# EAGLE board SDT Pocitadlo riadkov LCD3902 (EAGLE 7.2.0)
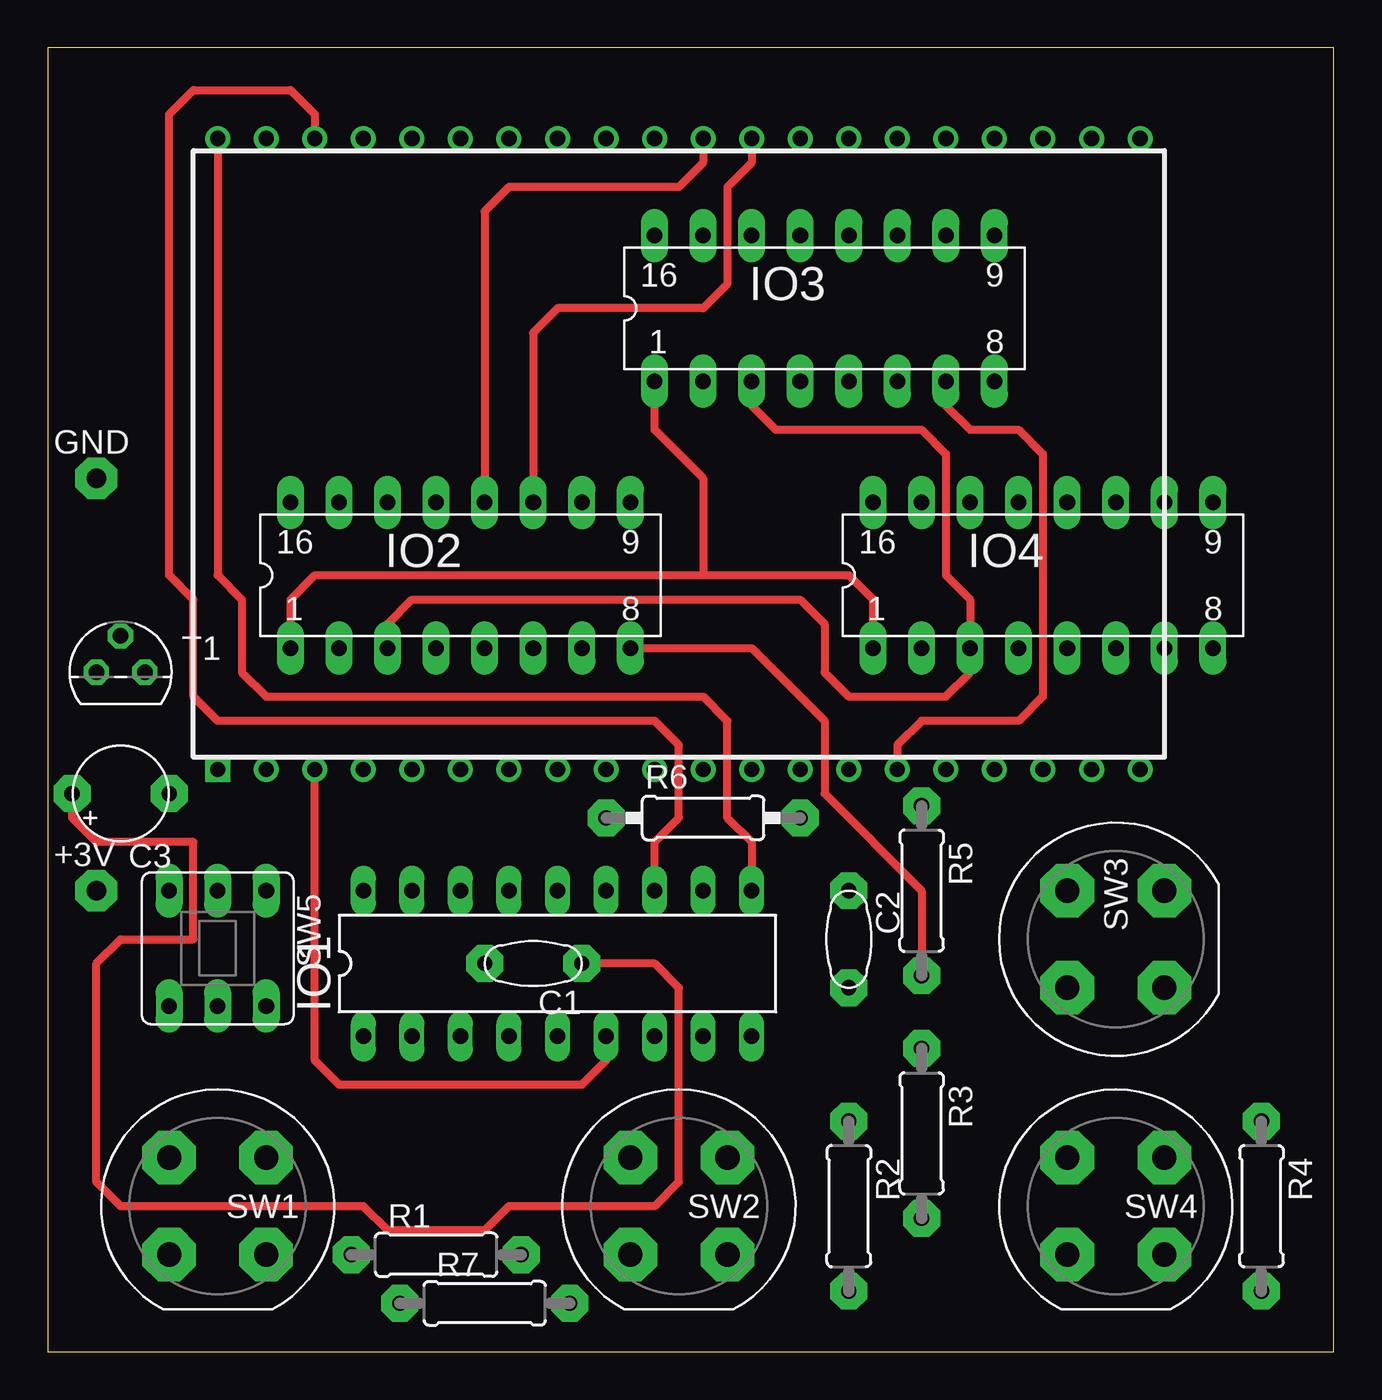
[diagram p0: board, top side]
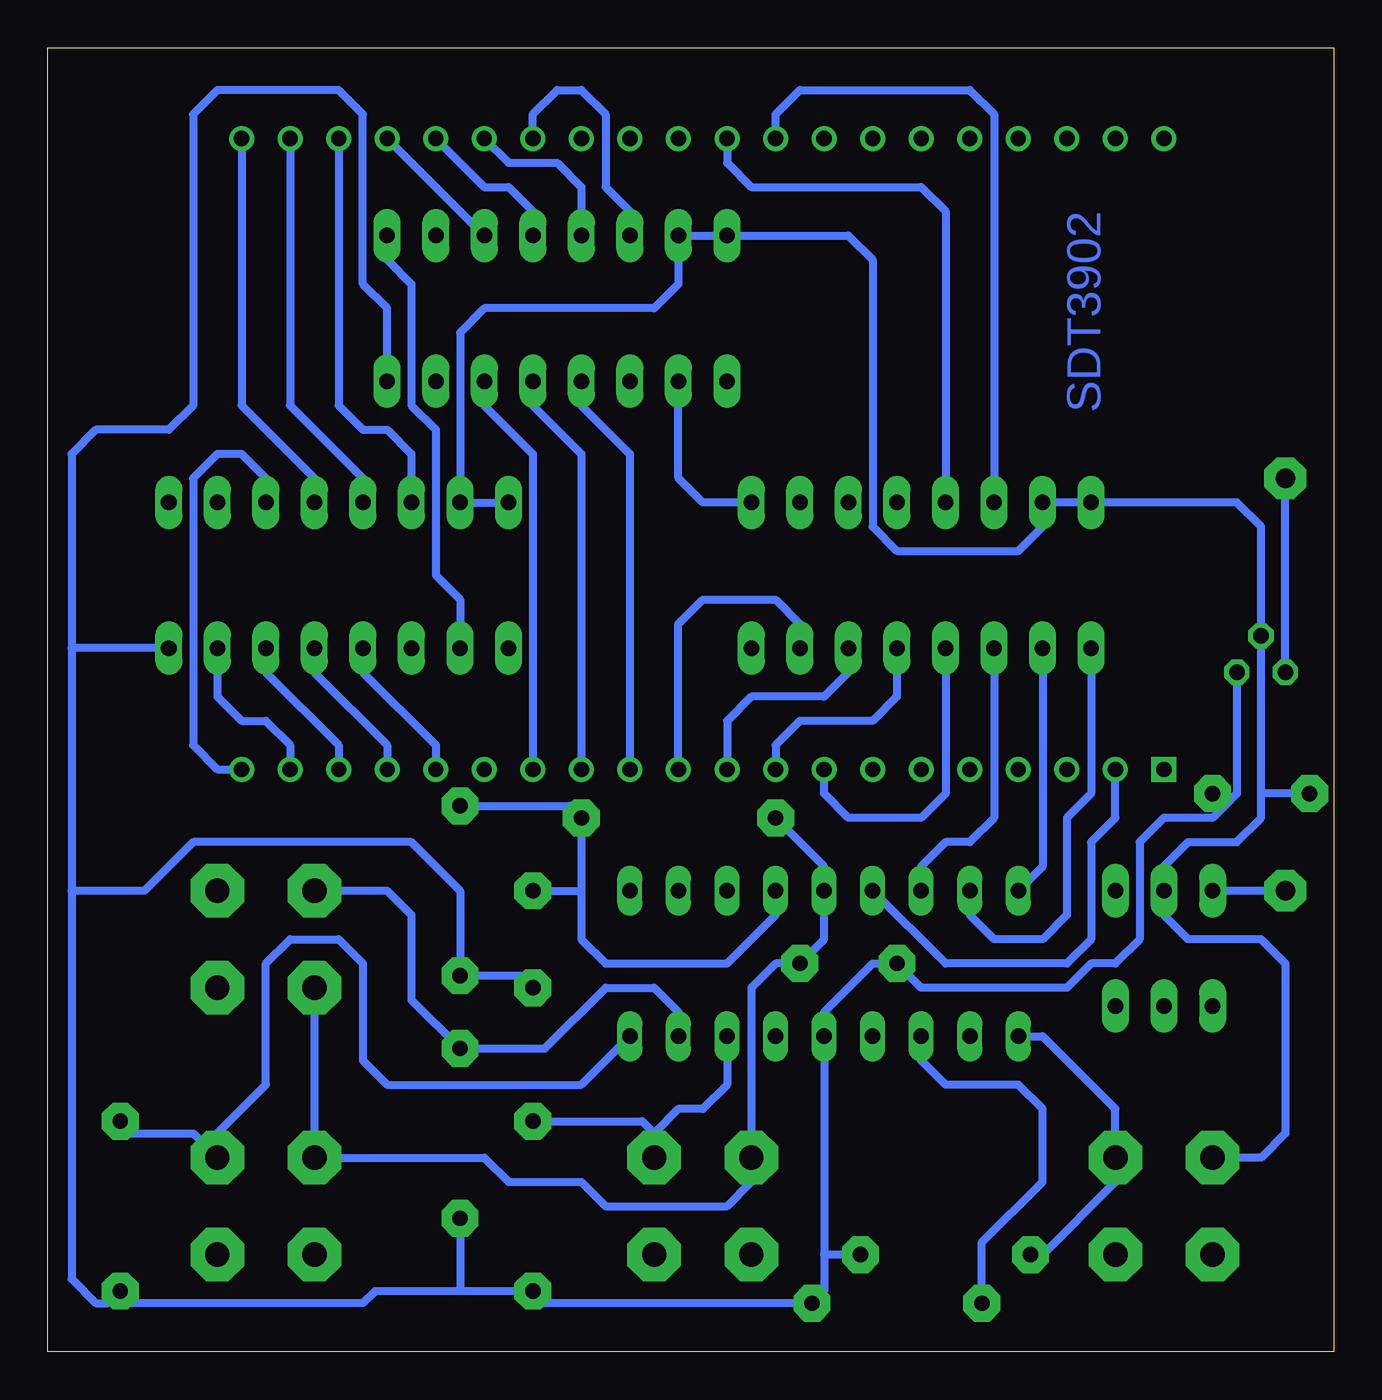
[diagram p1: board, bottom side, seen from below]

Size 67.29 x 68.25 mm. Coordinates in mm from the lower left corner, seen from the top.
Outline: 0,0 67.29,0 67.29,68.25 0,68.25 0,0
Copper layers (1*16): Top 0.035mm / dielectric 1.5mm / Bottom 0.035mm
Design rules "default": minimum track width 10mil, minimum drill 24mil, track to track 8mil, track to pad 8mil, pad to pad 8mil, via to via 8mil, smd to smd 8mil, copper to edge 40mil, drill to drill 8mil, minimum pad ring 10mil, minimum via ring 8mil, stop-mask expansion 4mil, vias tented up to drill 0mil, thermal gap 10mil

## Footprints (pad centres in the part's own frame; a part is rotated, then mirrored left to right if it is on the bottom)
PAD_1 = drill 1.016 pad 2.184 octagon: 1 0,0
KERAMICKY_RM5 = drill 0.8 pad 1.93 octagon: P$1 -2.54,0; P$2 2.54,0
ELEKTROLITICKY_RM5-5 = drill 0.8 pad 1.93 octagon: P$1 -2.54,0; P$2 2.54,0
4DR821_CN = drill 0.8 square: 1 -24.13,-16.51 | drill 0.8: 2 -21.59,-16.51; 3 -19.05,-16.51; 4 -16.51,-16.51; 5 -13.97,-16.51; 6 -11.43,-16.51; 7 -8.89,-16.51; 8 -6.35,-16.51; 9 -3.81,-16.51; 10 -1.27,-16.51; 11 1.27,-16.51; 12 3.81,-16.51; 13 6.35,-16.51; 14 8.89,-16.51; 15 11.43,-16.51; 16 13.97,-16.51; 17 16.51,-16.51; 18 19.05,-16.51; 19 21.59,-16.51; 20 24.13,-16.51; 21 24.13,16.51; 22 21.59,16.51; 23 19.05,16.51; 24 16.51,16.51; 25 13.97,16.51; 26 11.43,16.51; 27 8.89,16.51; 28 6.35,16.51; 29 3.81,16.51; 30 1.27,16.51; 31 -1.27,16.51; 32 -3.81,16.51; 33 -6.35,16.51; 34 -8.89,16.51; 35 -11.43,16.51; 36 -13.97,16.51; 37 -16.51,16.51; 38 -19.05,16.51; 39 -21.59,16.51; 40 -24.13,16.51
DIL18 = drill 0.813 long: 1 -8.89,-3.81; 2 -6.35,-3.81; 3 -3.81,-3.81; 4 -1.27,-3.81; 5 1.27,-3.81; 6 3.81,-3.81; 7 6.35,-3.81; 8 8.89,-3.81; 9 11.43,-3.81; 10 11.43,3.81; 11 8.89,3.81; 12 6.35,3.81; 13 3.81,3.81; 14 1.27,3.81; 15 -1.27,3.81; 16 -3.81,3.81; 17 -6.35,3.81; 18 -8.89,3.81
DIL16 = drill 0.813 pad 1.4 long: 1 -8.89,-3.81; 2 -6.35,-3.81; 3 -3.81,-3.81; 4 -1.27,-3.81; 5 1.27,-3.81; 6 3.81,-3.81; 7 6.35,-3.81; 8 8.89,-3.81; 9 8.89,3.81; 10 6.35,3.81; 11 3.81,3.81; 12 1.27,3.81; 13 -1.27,3.81; 14 -3.81,3.81; 15 -6.35,3.81; 16 -8.89,3.81
0207/7 = drill 0.8 pad 1.93 octagon: 1 -4.445,0; 2 4.445,0
0207/10 = drill 0.8 pad 1.93 octagon: 1 -5.08,0; 2 5.08,0
P-DT6 = drill 1.27 pad 2.8 octagon: 1 -2.54,-2.54; 1A -2.54,2.54; 2 2.54,-2.54; 2A 2.54,2.54
P-B170 = drill 0.813 pad 1.4 long: 1 0,5.08; 2 0,2.54; 3 0,0; 4 6.032,0; 5 6.032,2.54; 6 6.032,5.08
TO92 = drill 0.813 octagon: 1 1.27,0; 2 0,1.905; 3 -1.27,0

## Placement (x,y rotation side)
+3V  +3V  [PAD_1]  2.54,24.13 0 top
C1  100nF  [KERAMICKY_RM5]  25.4,20.32 180 top
C2  100nF  [KERAMICKY_RM5]  41.91,21.59 270 top
C3  100uF  [ELEKTROLITICKY_RM5-5]  3.81,29.21 180 top
DISPLAY  LCD3902  [4DR821_CN]  33.02,46.99 0 top
GND  GND  [PAD_1]  2.54,45.72 0 top
IO1  18M2  [DIL18]  25.4,20.32 0 top
IO2  4094  [DIL16]  21.59,40.64 0 top
IO3  4094  [DIL16]  40.64,54.61 0 top
IO4  4094  [DIL16]  52.07,40.64 0 top
R1  15K  [0207/7]  20.32,5.08 0 top
R2  15K  [0207/7]  41.91,7.62 270 top
R3  15K  [0207/7]  45.72,11.43 270 top
R4  15K  [0207/7]  63.5,7.62 270 top
R5  1K1  [0207/7]  45.72,24.13 270 top
R6  10K  [0207/10]  34.29,27.94 0 top
R7  15K  [0207/7]  22.86,2.54 0 top
SW1  DEL/BAT  [P-DT6]  8.89,7.62 180 top
SW2  PRG  [P-DT6]  33.02,7.62 180 top
SW3  UP  [P-DT6]  55.88,21.59 270 top
SW4  DOWN  [P-DT6]  55.88,7.62 180 top
SW5  P-B170  [P-B170]  6.35,24.13 270 top
T1  2N7000  [TO92]  3.81,35.56 0 top

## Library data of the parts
+3V GND = #PaJa_32
C1-C3 = #Kondenzatory
DISPLAY = 4DR821
IO1 = picaxe-4
IO2-IO4 = #PaJa_92
R1-R7 = #Odpory
SW1-SW4 = #PaJa_16
SW5 = #PaJa_prepinace
T1 = transistor-fet

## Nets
N$1: DISPLAY.16 IO4.4
N$2: DISPLAY.17 IO4.5
N$3: DISPLAY.18 IO4.6
N$4: DISPLAY.19 IO4.7
N$5: DISPLAY.20 IO4.11
N$6: DISPLAY.21 IO4.12
N$7: DISPLAY.22 IO4.13
N$8: DISPLAY.23 IO4.14
N$9: DISPLAY.24 IO3.11
N$10: DISPLAY.25 IO3.12
N$11: DISPLAY.26 IO3.13
N$12: DISPLAY.27 IO3.14
N$13: IO3.9 IO4.2
N$14: IO1.16 IO2.3 IO3.3 IO4.3
N$15: IO1.17 IO2.1 IO3.1 IO4.1
N$16: C1.P$2 C2.P$2 C3.P$1 IO1.5 IO2.8 IO3.8 IO4.8 R1.2 R2.2 R3.2 R4.2 R5.2 R7.2 T1.1
N$17: C2.P$1 IO1.13 R5.1 R6.2
N$18: DISPLAY.2 IO1.15
N$19: DISPLAY.40 IO1.10
N$20: DISPLAY.38 IO1.12
N$21: IO2.9 IO3.2
N$22: IO1.18 IO2.2
N$23: DISPLAY.12 IO3.4
N$24: DISPLAY.3 IO1.6
N$25: DISPLAY.8 IO2.4
N$26: DISPLAY.9 IO2.5
N$27: DISPLAY.10 IO2.6
N$28: DISPLAY.13 IO3.5
N$29: DISPLAY.14 IO3.6
N$30: DISPLAY.15 IO3.7
N$31: DISPLAY.32 IO2.14
N$32: DISPLAY.31 IO2.13
N$33: DISPLAY.30 IO2.12
N$34: DISPLAY.29 IO2.11
N$35: DISPLAY.11 IO2.7
N$36: IO1.1 R1.1 SW1.1
N$37: IO1.7 R2.1 SW2.1
N$38: IO1.8 R3.1 SW3.1
N$39: IO1.9 R4.1 SW4.1
N$40: C1.P$1 C3.P$2 IO1.14 IO2.15 IO2.16 IO3.15 IO3.16 IO4.15 IO4.16 R6.1 SW1.2 SW2.2 SW3.2 SW4.2 SW5.2 T1.2
N$41: GND.1 T1.3
N$42: +3V.1 SW5.3
N$43: IO1.3 R7.1

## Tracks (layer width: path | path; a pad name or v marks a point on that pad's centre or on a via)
N$1
  Bottom 0.406: IO4.4 50.8,35.56 46.99,31.75 DISPLAY.16
N$2
  Bottom 0.406: IO4.5 53.34,35.56 49.53,31.75 DISPLAY.17
N$3
  Bottom 0.406: IO4.6 55.88,35.56 52.07,31.75 DISPLAY.18
N$4
  Bottom 0.406: IO4.7 58.42,34.29 57.15,33.02 55.88,33.02 54.61,31.75 DISPLAY.19
N$5
  Bottom 0.406: IO4.11 55.88,45.72 57.15,46.99 58.42,46.99 59.69,45.72 59.69,31.75 58.42,30.48 DISPLAY.20
N$6
  Bottom 0.406: DISPLAY.21 57.15,49.53 53.34,45.72 IO4.12
N$7
  Bottom 0.406: DISPLAY.22 54.61,49.53 50.8,45.72 IO4.13
N$8
  Bottom 0.406: DISPLAY.23 52.07,49.53 50.8,48.26 49.53,48.26 48.26,46.99 IO4.14
N$9
  Bottom 0.406: DISPLAY.24 IO3.11
N$10
  Bottom 0.406: DISPLAY.25 44.45,60.96 43.18,60.96 41.91,59.69 IO3.12
N$11
  Bottom 0.406: DISPLAY.26 43.18,62.23 40.64,62.23 39.37,60.96 IO3.13
N$12
  Bottom 0.406: DISPLAY.27 41.91,64.77 40.64,66.04 39.37,66.04 38.1,64.77 38.1,60.96 36.83,59.69 IO3.14
N$13
  Bottom 0.406: IO3.9 49.53,57.15 48.26,55.88 48.26,49.53 46.99,48.26 46.99,40.64 45.72,39.37 IO4.2
N$14
  Top 0.406: IO2.3 17.78,38.1 19.05,39.37 39.37,39.37 40.64,38.1 40.64,35.56 41.91,34.29 46.99,34.29 48.26,35.56 IO4.3 48.26,39.37 46.99,40.64 46.99,46.99 45.72,48.26 38.1,48.26 36.83,49.53 IO3.3
  Bottom 0.406: IO2.3 17.78,27.94 19.05,26.67 20.32,26.67 21.59,25.4 IO1.16
N$15
  Top 0.406: IO2.1 12.7,39.37 13.97,40.64 34.29,40.64 | 34.29,40.64 41.91,40.64 43.18,39.37 IO4.1 | IO3.1 31.75,48.26 34.29,45.72 34.29,40.64
  Bottom 0.406: IO2.1 12.7,29.21 13.97,27.94 13.97,22.86 15.24,21.59 17.78,21.59 19.05,22.86 IO1.17
N$16
  Top 0.406: R5.2 45.72,24.13 40.64,29.21 40.64,33.02 36.83,36.83 IO2.8
  Bottom 0.406: T1.1 5.08,29.21 5.71,28.57 | 5.71,28.57 6.35,27.94 8.89,27.94 10.16,26.67 10.16,21.59 11.43,20.32 12.7,20.32 13.97,19.05 21.59,19.05 C1.P$2 24.13,20.32 26.67,17.78 IO1.5 26.67,5.08 | 45.72,3.17 R2.2 41.27,2.54 R7.2 26.67,3.17 26.67,5.08 | 45.72,3.17 50.16,3.17 50.8,2.54 62.87,2.54 R4.2 64.14,2.54 64.77,2.54 66.04,3.81 66.04,24.13 | R3.2 45.72,3.17 | IO4.8 66.04,36.83 | 66.04,36.83 66.04,24.13 | IO3.8 49.53,54.61 50.8,55.88 50.8,64.77 52.07,66.04 58.42,66.04 59.69,64.77 59.69,49.53 60.96,48.26 64.77,48.26 66.04,46.99 66.04,36.83 | C2.P$2 42.55,19.68 R5.2 45.72,24.13 48.26,26.67 59.69,26.67 62.23,24.13 66.04,24.13 | C3.P$1 5.71,28.57 | R1.2 26.67,5.08
N$17
  Bottom 0.406: 39.37,24.13 R6.2 40.01,28.57 R5.1 | 39.37,24.13 39.37,21.59 38.1,20.32 31.75,20.32 29.21,22.86 IO1.13 | C2.P$1 39.37,24.13
N$18
  Bottom 0.406: IO1.15 20.32,20.32 13.97,20.32 12.7,21.59 12.7,26.67 11.43,27.94 DISPLAY.2
N$19
  Top 0.406: IO1.10 36.83,26.67 35.56,27.94 35.56,33.02 34.29,34.29 11.43,34.29 10.16,35.56 10.16,39.37 8.89,40.64 DISPLAY.40
N$20
  Top 0.406: DISPLAY.38 13.97,64.77 12.7,66.04 7.62,66.04 6.35,64.77 6.35,40.64 7.62,39.37 7.62,34.29 8.89,33.02 31.75,33.02 33.02,31.75 33.02,27.94 31.75,26.67 IO1.12
N$21
  Bottom 0.406: IO2.9 33.02,44.45 34.29,45.72 IO3.2
N$22
  Bottom 0.406: IO2.2 15.24,25.4 IO1.18
N$23
  Bottom 0.406: IO3.4 39.37,49.53 36.83,46.99 DISPLAY.12
N$24
  Top 0.406: IO1.6 29.21,15.24 27.94,13.97 15.24,13.97 13.97,15.24 DISPLAY.3
N$25
  Bottom 0.406: IO2.4 20.32,29.21 21.59,27.94 25.4,27.94 26.67,29.21 DISPLAY.8
N$26
  Bottom 0.406: IO2.5 22.86,34.29 24.13,33.02 27.94,33.02 29.21,31.75 DISPLAY.9
N$27
  Bottom 0.406: IO2.6 25.4,35.56 26.67,34.29 30.48,34.29 31.75,33.02 DISPLAY.10
N$28
  Bottom 0.406: IO3.5 41.91,49.53 39.37,46.99 DISPLAY.13
N$29
  Bottom 0.406: IO3.6 44.45,49.53 41.91,46.99 DISPLAY.14
N$30
  Top 0.406: IO3.7 46.99,49.53 48.26,48.26 50.8,48.26 52.07,46.99 52.07,34.29 50.8,33.02 45.72,33.02 44.45,31.75 DISPLAY.15
N$31
  Bottom 0.406: DISPLAY.32 29.21,64.77 27.94,66.04 19.05,66.04 17.78,64.77 IO2.14
N$32
  Bottom 0.406: DISPLAY.31 31.75,62.23 30.48,60.96 21.59,60.96 20.32,59.69 IO2.13
N$33
  Top 0.406: DISPLAY.30 34.29,62.23 33.02,60.96 24.13,60.96 22.86,59.69 IO2.12
N$34
  Top 0.406: DISPLAY.29 36.83,62.23 35.56,60.96 35.56,55.88 34.29,54.61 26.67,54.61 25.4,53.34 IO2.11
N$35
  Bottom 0.406: DISPLAY.11 34.29,38.1 33.02,39.37 29.21,39.37 27.94,38.1 IO2.7
N$36
  Bottom 0.406: IO1.1 15.24,16.51 11.43,12.7 SW1.1 11.43,8.89 15.24,5.08 R1.1
N$37
  Bottom 0.406: IO1.7 31.75,13.97 33.02,12.7 34.29,12.7 35.56,11.43 | 35.56,11.43 SW2.1 | R2.1 36.2,12.06 35.56,11.43
N$38
  Bottom 0.406: IO1.8 34.29,17.78 35.56,19.05 38.1,19.05 41.27,15.88 R3.1 48.26,18.41 48.26,22.86 49.53,24.13 SW3.1
N$39
  Bottom 0.406: R4.1 63.5,11.43 59.69,11.43 SW4.1 58.42,11.43 55.88,13.97 55.88,20.32 54.61,21.59 52.07,21.59 50.8,20.32 50.8,15.24 49.53,13.97 39.37,13.97 IO1.9
N$40
  Top 0.406: C1.P$1 31.75,20.32 33.02,19.05 33.02,8.89 31.75,7.62 24.13,7.62 22.86,6.35 17.78,6.35 16.51,7.62 3.81,7.62 2.54,8.89 2.54,20.32 3.81,21.59 7.62,21.59 7.62,26.67 2.54,26.67 1.27,27.94 C3.P$2
  Bottom 0.406: SW1.2 3.81,10.16 2.54,11.43 2.54,20.32 3.81,21.59 7.62,21.59 8.89,22.86 SW5.2 8.89,25.4 7.62,26.67 5.08,26.67 3.81,27.94 3.81,29.21 | IO4.16 IO4.15 45.72,53.34 44.45,54.61 35.56,54.61 34.29,55.88 IO3.15 IO3.16 25.4,58.42 24.13,57.15 24.13,43.18 22.86,41.91 16.51,41.91 15.24,43.18 IO2.15 IO2.16 5.08,44.45 3.81,43.18 T1.2 3.81,29.21 | R6.1 26.67,25.4 IO1.14 26.67,21.59 C1.P$1 29.21,20.32 30.48,19.05 SW2.2 30.48,8.89 31.75,7.62 38.1,7.62 39.37,8.89 43.18,8.89 44.45,10.16 SW4.2 SW3.2 | C3.P$2 3.81,29.21
N$41
  Bottom 0.406: T1.3 GND.1
N$42
  Bottom 0.406: +3V.1 SW5.3
N$43
  Bottom 0.406: IO1.3 21.59,15.24 20.32,13.97 16.51,13.97 15.24,12.7 15.24,8.89 18.41,5.71 R7.1

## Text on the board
Bottom: SDT3902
